VAR_GLOBAL

stButtons : ST_Buttons;

{attribute 'TcLinkTo':='TIID^Device 2 (EtherCAT)^Term 1 (EK1200)^Term 6 (EL6090)^DIS Inputs^Status^Up'}
IgbUp AT %I* : BOOL;

{attribute 'TcLinkTo':='TIID^Device 2 (EtherCAT)^Term 1 (EK1200)^Term 6 (EL6090)^DIS Inputs^Status^Down'}
IgbDown AT %I* : BOOL;

{attribute 'TcLinkTo':='TIID^Device 2 (EtherCAT)^Term 1 (EK1200)^Term 6 (EL6090)^DIS Inputs^Status^Left'}
IgbLeft AT %I* : BOOL;

{attribute 'TcLinkTo':='TIID^Device 2 (EtherCAT)^Term 1 (EK1200)^Term 6 (EL6090)^DIS Inputs^Status^Right'}
IgbRight AT %I* : BOOL;

{attribute 'TcLinkTo':='TIID^Device 2 (EtherCAT)^Term 1 (EK1200)^Term 6 (EL6090)^DIS Inputs^Status^Enter'}
IgbEnter AT %I* : BOOL;


END_VAR
